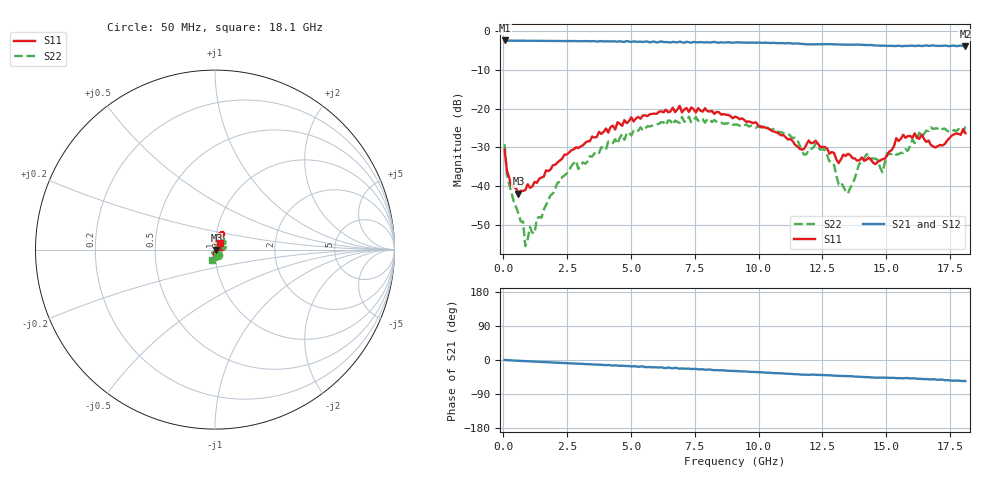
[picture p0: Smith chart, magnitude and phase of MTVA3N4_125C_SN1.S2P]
! Network Analyzer HP8720D.06.14 Serial No. US36140669
! 27 Jun 2005  09:47:17
! Frequency  S11  S21  S12  S22
# HZ  S  DB R 50
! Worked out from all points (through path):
!   201 points, 50 MHz to 18.1 GHz, reference 50 ohm
!   highest |S21| = -2.36 dB at 50 MHz (marker M1); lowest = -3.9 dB at 18.1 GHz (marker M2)
!   group delay of S21, straight-line fit = 8.5 ps
!   lowest |S11| = -41.9 dB at 591.5 MHz (marker M3), VSWR 1.02, Z = 50.8 - j0.215 ohm
!   |S11| at or under -10 dB: start of sweep to end of sweep
!   |S22| runs from -55.5 to -22.0 dB; largest |S21 - S12| = 0.022
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5e7  -30.61 -64.0  -2.36 0.1  -2.41 0.5  -29.16 -59.5
1.4025e8  -35.95 -54.5  -2.45 -0.3  -2.43 -0.3  -37.04 -68.6
5.915e8  -41.91 -15.3  -2.42 -1.9  -2.44 -1.9  -47.09 -38.6
7.72e8  -41.25 -0.8  -2.43 -2.8  -2.42 -2.6  -49.15 -35.4
8.6225e8  -40.98 -1.8  -2.44 -2.9  -2.45 -2.9  -55.49 -35.3
1.04275e9  -40.42 12.2  -2.44 -3.7  -2.44 -3.5  -50.54 0.4
2.12575e9  -33.84 28.0  -2.48 -7.2  -2.49 -7.2  -39.08 66.8
3.1185e9  -29.44 41.5  -2.53 -10.1  -2.55 -10.4  -33.86 75.0
6.09675e9  -20.77 61.3  -2.74 -19.9  -2.67 -19.9  -23.88 55.0
9.075e9  -22.05 78.1  -2.88 -29.0  -2.86 -29.2  -24.07 24.2
1.115075e10  -27.93 82.2  -3.03 -36.4  -3.08 -36.7  -26.44 9.8
1.169225e10  -30.59 91.7  -3.26 -38.8  -3.26 -38.8  -30.90 14.3
1.21435e10  -28.75 78.6  -3.39 -38.4  -3.36 -38.7  -30.04 40.9
1.259475e10  -29.91 60.9  -3.36 -39.8  -3.34 -39.8  -30.72 36.7
1.313625e10  -34.03 42.9  -3.43 -41.8  -3.39 -42.1  -39.55 6.0
1.349725e10  -31.63 20.8  -3.47 -42.8  -3.45 -42.8  -41.90 -54.5
1.421925e10  -33.21 -16.3  -3.56 -44.9  -3.55 -45.2  -31.77 -122.8
1.4851e10  -33.04 -1.8  -3.73 -46.8  -3.68 -46.7  -36.45 -108.1
1.512175e10  -31.07 8.9  -3.77 -47.3  -3.71 -47.2  -31.62 -99.8
1.566325e10  -26.72 2.1  -3.83 -48.5  -3.75 -47.8  -31.43 -91.3
1.674625e10  -29.34 8.9  -3.72 -51.4  -3.85 -51.3  -24.77 -77.2
1.81e10  -26.34 50.9  -3.92 -55.6  -3.88 -56.5  -24.60 -107.3
